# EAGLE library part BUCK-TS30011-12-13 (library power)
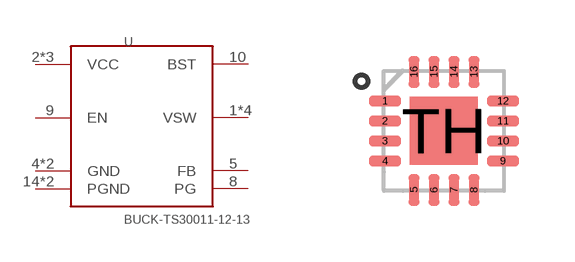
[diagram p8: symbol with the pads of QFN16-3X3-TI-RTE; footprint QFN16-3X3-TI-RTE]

Designator prefix U

## BUCK-TS30011-12-13QFN  [QFN16-3X3-TI-RTE]
1  VSW
2  VCC
3  VCC
4  GND
5  FB
8  PG
9  EN
10  BST
11  VCC
12  VSW
13  VSW
14  PGND
15  PGND
16  VSW
TH  GND

## Footprint QFN16-3X3-TI-RTE (pad centres in mm)
3x3 mm
smd 0.8 x 0.275: 1 -1.475,0.75; 2 -1.475,0.25; 3 -1.475,-0.25; 4 -1.475,-0.75; 9 1.475,-0.75; 10 1.475,-0.25; 11 1.475,0.25; 12 1.475,0.75
smd 0.275 x 0.8: 5 -0.75,-1.475; 6 -0.25,-1.475; 7 0.25,-1.475; 8 0.75,-1.475; 13 0.75,1.475; 14 0.25,1.475; 15 -0.25,1.475; 16 -0.75,1.475
smd 1.7 x 1.7: TH 0,0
